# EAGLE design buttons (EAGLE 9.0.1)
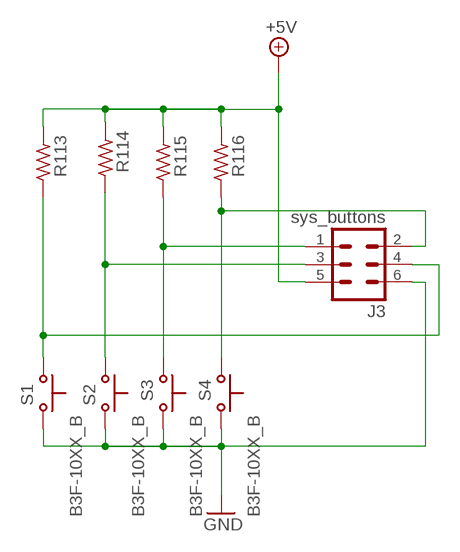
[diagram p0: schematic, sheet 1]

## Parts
J3  sys_buttons  MA03-2  [MA03-2]
R113  R-EU_0204/7  [0204/7]
R114  R-EU_0204/7  [0204/7]
R115  R-EU_0204/7  [0204/7]
R116  R-EU_0204/7  [0204/7]
S1  B3F-10XX_B  [B3F-10XX_B]
S2  B3F-10XX_B  [B3F-10XX_B]
S3  B3F-10XX_B  [B3F-10XX_B]
S4  B3F-10XX_B  [B3F-10XX_B]

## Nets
+5V: J3.5 R113.1 R114.1 R115.1 R116.1
GND: J3.6 S1.3(S) S1.4(S) S2.3(S) S2.4(S) S3.3(S) S3.4(S) S4.3(S) S4.4(S)
S1: J3.4 R113.2 S1.1(P) S1.2(P)
S2: J3.3 R114.2 S2.1(P) S2.2(P)
S3: J3.1 R115.2 S3.1(P) S3.2(P)
S4: J3.2 R116.2 S4.1(P) S4.2(P)

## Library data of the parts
J3 = con-lstb:MA03-2: PIN HEADER
R113-R116 = rcl:R-EU_: RESISTOR, European symbol
S1-S4 = switch-omron:B3F-10XX: Tactile Switch

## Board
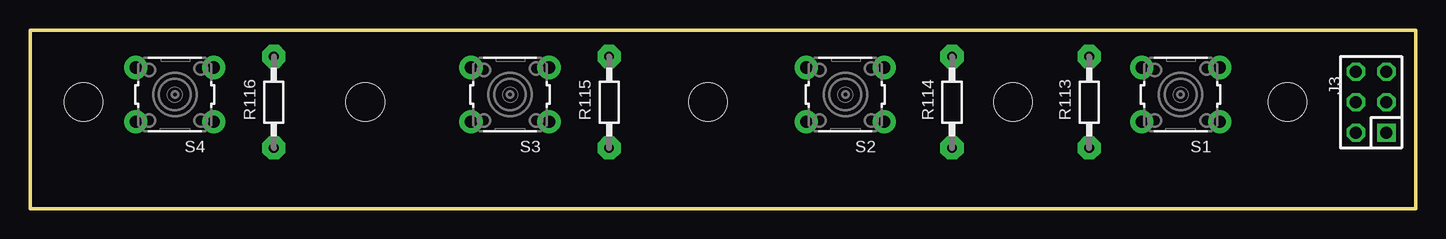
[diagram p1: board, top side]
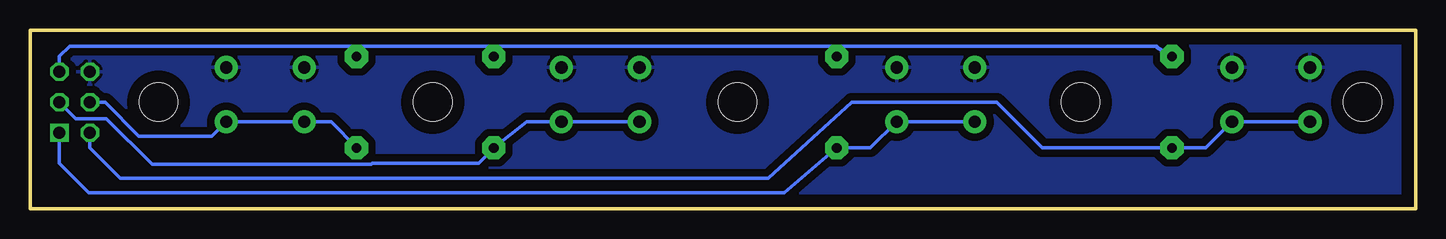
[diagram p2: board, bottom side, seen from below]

Size 115.48 x 14.91 mm. Coordinates in mm from the lower left corner, seen from the top.
Outline: 115.48,0 115.48,14.91 0,14.91 0,0 115.48,0
Copper layers (1*16): Top 0.035mm / dielectric 1.5mm / Bottom 0.035mm
Design rules "default": minimum track width 10mil, minimum drill 24mil, track to track 8mil, track to pad 8mil, pad to pad 8mil, via to via 8mil, smd to smd 8mil, copper to edge 40mil, drill to drill 8mil, minimum pad ring 10mil, minimum via ring 8mil, stop-mask expansion 4mil, vias tented up to drill 0mil, thermal gap 10mil
Holes 3.2 mm at 4.45,8.89 56.52,8.89 104.78,8.89 27.94,8.89 81.92,8.89

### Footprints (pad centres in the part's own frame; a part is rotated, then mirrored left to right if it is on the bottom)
MA03-2 = drill 1.016 square: 1 -2.54,-1.27 | drill 1.016 octagon: 2 -2.54,1.27; 3 0,-1.27; 4 0,1.27; 5 2.54,-1.27; 6 2.54,1.27
0204/7 = drill 0.813 pad 1.93 octagon: 1 -3.81,0; 2 3.81,0
B3F-10XX_B = drill 1.016 pad 1.93: 1 -3.251,2.261; 2 3.251,2.261; 3 -3.251,-2.261; 4 3.251,-2.261

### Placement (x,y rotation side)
J3  111.76,8.89 90 top
R113  88.27,8.89 270 top
R114  76.83,8.89 270 top
R115  48.26,8.89 270 top
R116  20.32,8.89 270 top
S1  95.89,9.53 180 top
S2  67.94,9.53 180 top
S3  40.01,9.53 180 top
S4  12.06,9.53 180 top

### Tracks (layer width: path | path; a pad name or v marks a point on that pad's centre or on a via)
+5V
  Bottom 0.305: J3.5 113.03,12.7 112.17,13.56 88.27,13.56 | 48.35,13.56 R115.1 | 88.27,13.56 76.2,13.56 | 76.2,13.56 48.35,13.56 | R114.1 76.2,13.56 | R113.1 88.27,13.56 | R116.1 21.59,13.46 21.59,13.56 48.35,13.56
GND
  Bottom 0.305: S3.3 43.54,12.07
  pour Bottom (isolate 0.61): 115.49,0 115.49,14.68 0.08,14.68 0.08,0
S1
  Bottom 0.305: J3.4 109.22,8.89 106.4,6.07 100.33,6.07 S1.1 S1.2 90.4,7.26 R113.2
S2
  Bottom 0.305: S2.2 S2.1 74.07,7.26 R114.2 78.11,3.81 86.96,3.81 87.06,3.71 105.31,3.71 109.12,7.52 111.66,7.52 J3.3
S3
  Bottom 0.305: S3.2 S3.1 45.44,5.08 R115.2 52.63,1.35 110.57,1.35 113.03,3.81 J3.1
S4
  Bottom 0.305: S4.2 S4.1 17.5,5.08 R116.2 31.11,5.08 34.92,8.89 46.99,8.89 53.98,2.54 107.95,2.54 110.49,5.08 J3.2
